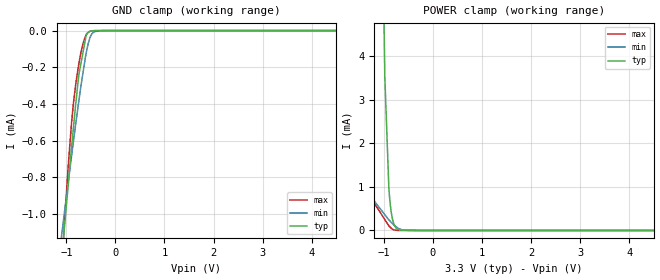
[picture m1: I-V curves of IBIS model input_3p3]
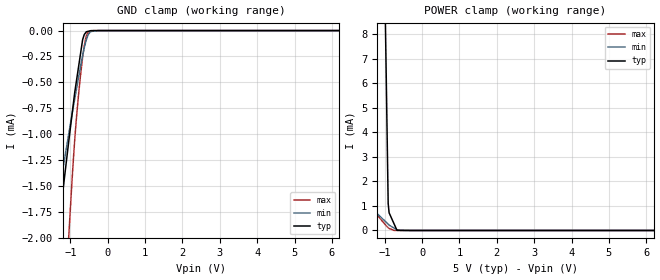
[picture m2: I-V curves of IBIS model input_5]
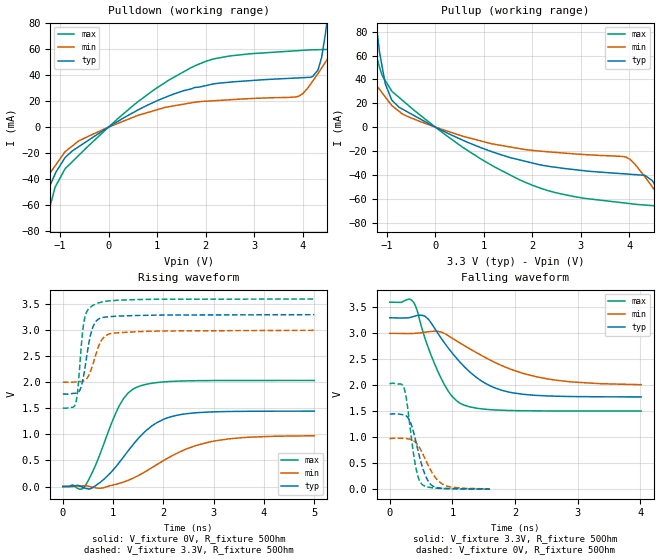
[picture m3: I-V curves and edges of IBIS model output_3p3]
|Texas Instruments Incorporated
| 10MHz Modulator with built in current excitation for Hall sensors
| Marketing part#   Digital Voltage Range   Package-type   #pins
| ADS1208IPW   2.7V - 5.5V   TSSOP   16
| ADS1208IPWG4   2.7V - 5.5V   TSSOP   16
| ADS1208IPWR   2.7V - 5.5V   TSSOP   16
| ADS1208IPWRG4   2.7V - 5.5V   TSSOP   16
[IBIS Ver]   3.2
[File name]   ads1208.ibs
|SIMDE Ver   V3.0 - 201101 - RHL4 - Build 457
[File Rev]   1.0
[Date]   5/16/2011
[Source]
| Texas Instruments Incorporated.
| Analog-eLab Design Center, HPA
| 12500 TI Blvd
| Dallas, TX -75243
| e-mail: elab_ibis@list.ti.com
[Notes]   Revision History:
| Rev 1.0: 5/16/2011
| - Initial version of the model
| - Model generated from simulations in TISPICE
| - Model matched to SPICE simulation
| - C_comp although listed in numerical order of value are
|   obtained from varying PVT conditions. For PVT conditions for
|   each specific value refer the buffer description under
|   respective [Model]. IBIS model user is responsible for using
|   appropriate C_comp to simulate for Signal Integrity.
| - Model names with a trailing _3p3 contains the model for
|   3.3V [3.0V and 3.6V]. Model names with a trailing _5 contains
|   the model for 5.0V [4.5V and 5.5V].
[Disclaimer]
| This model is designed as an aid for customers of Texas Instruments.
| TI and its licensors and suppliers make no warranties, either expressed
| or implied, with respect to this  model, including the warranties of
| merchantability or fitness for a particular purpose. The model is
| provided solely on an "as is" basis. The entire risk as to its quality
| and performance is with the customer.
[Copyright]
 (C) Copyright 2011 Texas Instruments Incorporated.All rights reserved.
|   ADS1208
[Component]   ADS1208
[Manufacturer]   TI
[Package]   |16 TSSOP   -  PW package
|   typ   min   max
R_pkg   0.03926   0.03631   0.04323
L_pkg   2.65777nH   2.30021nH   3.16884nH
C_pkg   0.46553pF   0.42516pF   0.51250pF
[Pin]  signal_name   model_name   R_pin   L_pin   C_pin
1   IOUT   TERM   0.03861   3.16884nH  0.51250pF
2   IADJ   TERM   0.04306   2.75459nH  0.48880pF
3   AVDD   POWER   0.02116   2.08677nH  0.46132pF
4   VIN+   TERM   0.03638   2.30226nH  0.43259pF
5   VIN-   TERM   0.03822   2.36501nH  0.43620pF
6   AGND   GND   0.02283   2.19557nH  0.46635pF
7   REFIN   TERM   0.04323   2.76940nH  0.48912pF
8   REFOUT   TERM   0.03809   3.16350nH  0.51239pF
9   M1   INPUT   0.03770   3.14936nH  0.51152pF
10   M0   INPUT   0.04232   2.73683nH  0.48790pF
11   _MDATA   OUTPUT   0.03883   2.39107nH  0.42516pF
12   MDATA   OUTPUT   0.03631   2.30021nH  0.42953pF
13   _MCLK   MCLK_BAR   0.03697   2.32042nH  0.43088pF
14   MCLK   OUTPUT   0.04145   2.47181nH  0.42976pF
15   BGND   GND   0.04286   2.74791nH  0.48822pF
16   BVDD   POWER   0.03789   3.14597nH  0.51159pF
|   Model Selectors
[Model Selector] INPUT
input_3p3  3.3V digital input
input_5   5.0V digital input
[Model Selector] OUTPUT
output_3p3  3.3V digital output
output_5   5.0V digital output
[Model Selector] MCLK_BAR
mclk_bar_3p3  3.3V digital I/O
mclk_bar_5   5.0V digital I/O
[Model Selector] TERM
term_3-3V  3.3V nominal termination
term_5-0V  5.0V nominal termination
[Model] term_3-3V
Model_type Terminator
C_comp   1.0e-20F  1.0e-20F  1.0e-20F
|   typ   min   max
[Voltage Range]   3.3V   3.0V   3.6V
[POWER Clamp Reference]   3.3V   3.0V   3.6V
[GND Clamp Reference]   0V   0V   0V
|Ambient Temperature   25   85   -40
|Junction Temperature
[Temperature Range]   35   95   -40
[Model] term_5-0V
Model_type Terminator
C_comp   1.0e-20F  1.0e-20F  1.0e-20F
|   typ   min   max
[Voltage Range]   5.0V   4.5V   5.5V
[POWER Clamp Reference]   5.0V   4.5V   5.5V
[GND Clamp Reference]   0V   0V   0V
|Ambient Temperature   25   85   -40
|Junction Temperature
[Temperature Range]   35   95   -40
| Models and submodels in the file (8): input_3p3 (Input), input_5 (Input), output_3p3 (Output), output_5 (Output), mclk_bar_3p3 (I/O), mclk_bar_5 (I/O), term_3-3V (Terminator), term_5-0V (Terminator)
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|   input_3p3 Model
[Model]   input_3p3
Model_type   Input
Vinl = 0.8
Vinh = 2.0
|   typ   min   max
|   (nom PVT)   (fast PVT)   (slow PVT)
|C_comp from frequency sweep method (F=10MHz)
|Average
|C_comp   6.241e-13   5.507e-13   6.563e-13
|C_comp from LC tank measurement(L=1nH)
|Average
|Resonant Frequency(Hz)   5.262e+10   6.403e+10   7.720e+09
C_comp   9.157e-15   6.185e-15   4.254e-13
| Where nom  PVT is Nominal Process, 3.3V, 35C
|   Fast PVT is Strong Process,  3.6V, -40C
|   Slow PVT is Weak Process,   3V, 95C
[Voltage Range]   3.3   3   3.6
|Ambient Temperature   25   85   -40
|Junction Temperature
[Temperature Range]   35   95   -40
[Power Clamp Reference]   3.3   3   3.6
[GND Clamp Reference]   0   0   0
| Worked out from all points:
|   GND clamp passes 1 mA (typ) near -1.01 V on its own axis
|   POWER clamp passes 1 mA (typ) near -0.90 V on its own axis
[GND Clamp]
|   Voltage   I(typ)   I(min)   I(max)
-3.3V     -8.305mA   -6.084mA   -13.52mA
-1.188V   -1.522mA   -1.315mA   -1.706mA
-1.048V   -1.099mA   -1.01mA    -1.087mA
-896.4mV  -643.4uA   -689uA     -511.2uA
-813.6mV  -412.9uA   -518.6uA   -302.1uA
-745.8mV  -241.2uA   -385.3uA   -182.8uA
-658.8mV  -116.1uA   -227uA     -69.11uA
-590.7mV  -18.21uA   -115.8uA   -22.97uA
-534.6mV  -5.388uA   -52.7uA    -6.77uA
-429mV    -393nA     -5.602uA   -329.7nA
-285mV    -260.1nA   -127.2nA   -169.2nA
6.6V      0A         0A         0A
[POWER Clamp]
|   Voltage   I(typ)   I(min)   I(max)
-3.3V     1.038A     4.406mA    5.171mA
-3V       885.5mA    3.863mA    4.508mA
-1.386V   105.8mA    991.9uA    1.005mA
-1.04V    8.055mA    448.9uA    354.1uA
-980.1mV  3.535mA    362.7uA    249.8uA
-897.6mV  969.7uA    243.1uA    104.9uA
-867.9mV  585uA      208.4uA    71.07uA
-851.4mV  436.9uA    189.2uA    52.7uA
-806.4mV  190.1uA    136.9uA    19.42uA
-745.8mV  50.64uA    82uA       5.864uA
-666.6mV  6.537uA    30.76uA    434.9nA
6.6V      0A         0A         0A
|   input_5 Model
[Model]   input_5
Model_type   Input
Vinl = 1.5
Vinh = 3.5
|   typ   min   max
|   (nom PVT)   (fast PVT)   (slow PVT)
|C_comp from frequency sweep method (F=10MHz)
|Average
|C_comp   5.579e-13   4.948e-13   6.238e-13
|C_comp from LC tank measurement(L=1nH)
|Average
|Resonant Frequency(Hz)   5.197e+10   6.383e+10   8.320e+09
C_comp   9.388e-15   6.223e-15   3.663e-13
| Where nom  PVT is Nominal Process, 5V, 35C
|   Fast PVT is Strong Process,  5.5V, -40C
|   Slow PVT is Weak Process,   4.5V, 95C
[Model Spec]
|Subparameter   typ   min   max
Vinh   3.5   3.15   3.85
Vinl   1.5   1.35   1.65
[Voltage Range]   5   4.5   5.5
|Ambient Temperature   25   85   -40
|Junction Temperature
[Temperature Range]   35   95   -40
[Power Clamp Reference]   5   4.5   5.5
[GND Clamp Reference]   0   0   0
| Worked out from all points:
|   GND clamp passes 1 mA (typ) near -1.02 V on its own axis
|   POWER clamp passes 1 mA (typ) near -0.90 V on its own axis
[GND Clamp]
|   Voltage   I(typ)   I(min)   I(max)
-5V       -13.84mA   -9.976mA   -29.85mA
-1.601V   -2.825mA   -2.233mA   -5.783mA
-1.373V   -2.099mA   -1.722mA   -4.208mA
-1.188V   -1.523mA   -1.315mA   -2.955mA
-1.045V   -1.083mA   -1.007mA   -2.016mA
-880mV    -596.4uA   -660.7uA   -1.053mA
-786.5mV  -371.2uA   -471.3uA   -650.6uA
-670mV    -90.54uA   -243uA     -260.2uA
-570mV    -11.61uA   -88.91uA   -51.87uA
-454.5mV  -1.103uA   -9.818uA   -7.056uA
-252mV    -268.3nA   -46.33nA   -34.87nA
10V       0A         0A         0A
[POWER Clamp]
|   Voltage   I(typ)   I(min)   I(max)
-5V       1.912A     7.552mA    8.964mA
-4.5V     1.654A     6.628mA    7.863mA
-1.665V   227.4mA    1.468mA    1.621mA
-1.375V   101.4mA    973.6uA    982.5uA
-1.14V    24.49mA    602.2uA    522.2uA
-957mV    6.273mA    335.6uA    189.5uA
-905mV    1.096mA    259.8uA    114.2uA
-880mV    720.8uA    223.4uA    82.72uA
-748mV    272.3uA    98.92uA    2.991uA
-670mV    7.189uA    29.51uA    2.679uA
-435mV    0A         3.245uA    1.739uA
10V       0A         0A         0A
|   output_3p3 Model
[Model]   output_3p3
Model_type   Output
Polarity   Non-Inverting
Vmeas = 1.65
Vref = 1.65
Cref = 30pF
Rref = 50
|   typ   min   max
|   (nom PVT)   (fast PVT)   (slow PVT)
|C_comp from frequency sweep method (F=10MHz)
|C_comp   2.140e-12   2.125e-12   2.174e-12
|ON state : BUFFER OUTPUT TURNED HIGH
|C_comp   2.140e-12   2.125e-12   2.174e-12
|OFF state: BUFFER OUTPUT TURNED LOW
|C_comp   2.055e-12   1.892e-12   2.087e-12
|C_comp from LC tank measurement(L=1nH)
|Resonant Frequency(Hz)   5.890e+09   6.040e+09   4.920e+09
C_comp   7.309e-13   6.950e-13   1.047e-12
|ON state : BUFFER OUTPUT TURNED HIGH
|Resonant Frequency(Hz)   5.890e+09   6.040e+09   4.920e+09
|C_comp   7.309e-13   6.950e-13   1.047e-12
|OFF state: BUFFER OUTPUT TURNED LOW
|Resonant Frequency(Hz)   5.960e+09   6.210e+09   5.000e+09
|C_comp   7.138e-13   6.575e-13   1.014e-12
| Where nom  PVT is Nominal Process, 3.3V, 35C
|   Fast PVT is Strong Process,  3.6V, -40C
|   Slow PVT is Weak Process,   3V, 95C
[Voltage Range]   3.3   3   3.6
|Ambient Temperature   25   85   -40
|Junction Temperature
[Temperature Range]   35   95   -40
[Pullup Reference]   3.3   3   3.6
[Pulldown Reference]   0   0   0
[Power Clamp Reference]   3.3   3   3.6
[GND Clamp Reference]   0   0   0
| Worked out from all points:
|   slope of the pulldown table from 0 to 0.495 V, typ, clamps not added: 45.5 ohm
|   slope of the pullup table from 0 to 0.495 V, typ, clamps not added: 51.2 ohm
|   falling waveform, V_fixture 3.3V, R_fixture 50Ohm: 20-80 % time 696ps typ, 1.05ns min, 421ps max; typ from 3.3 V to 1.78 V
|   rising waveform, V_fixture 0V, R_fixture 50Ohm: 20-80 % time 789ps typ, 1.15ns min, 521ps max; typ from 0 V to 1.45 V
|   rising waveform, V_fixture 3.3V, R_fixture 50Ohm: 20-80 % time 170ps typ, 217ps min, 120ps max; typ from 1.78 V to 3.3 V
|   falling waveform, V_fixture 0V, R_fixture 50Ohm: 20-80 % time 193ps typ, 260ps min, 140ps max; typ from 1.45 V to 0.004 V
[Pulldown]
|   Voltage   I(typ)   I(min)   I(max)
-3.3V     -235.7mA   -157.4mA   -409.3mA
-2.239V   -138.2mA   -94.86mA   -228.4mA
-1.494V   -69.65mA   -50.91mA   -104.6mA
-1.339V   -56.04mA   -42.39mA   -79.85mA
-896.4mV  -23.44mA   -18.92mA   -32.04mA
1.804V    30.54mA    19.28mA    47.49mA
3.918V    37.83mA    23.71mA    58.78mA
4.316V    43.89mA    41.12mA    59.47mA
4.496V    79.66mA    51.4mA     59.66mA
4.77V     187.5mA    67.5mA     62.15mA
4.918V    256.1mA    76.32mA    77.72mA
6.6V      1.096A     178.4mA    358.6mA
[Pullup]
|   Voltage   I(typ)   I(min)   I(max)
-3.3V     1.096A     160mA      409.7mA
-2.148V   510.7mA    90.38mA    215.2mA
-1.482V   191.2mA    50.08mA    102.7mA
-1.294V   112mA      39.22mA    71.39mA
-1.033V   36.28mA    25.3mA     38.94mA
-745.8mV  16.6mA     13.14mA    24.8mA
1.836V    -28.44mA   -18.71mA   -45.95mA
3.933V    -39.25mA   -25.19mA   -63.72mA
4.468V    -44.78mA   -49.97mA   -65.74mA
4.975V    -86.86mA   -79.66mA   -88.67mA
5.069V    -94.78mA   -85.15mA   -102.6mA
6.6V      -235.9mA   -175.1mA   -358.1mA
[Ramp]
R_load = 50
|   typ   min   max
dV/dt_r   0.868601/7.88674e-10   0.584928/1.15225e-09   1.22229/5.19124e-10
dV/dt_f   0.914229/6.96224e-10   0.596986/1.06545e-09   1.25642/4.21049e-10
[Falling Waveform]
V_fixture = 3.3V
V_fixture_min = 3V
V_fixture_max = 3.6V
R_fixture = 50Ohm
|   Time   V(typ)   V(min)   V(max)
0s        3.3V       3V         3.6V
378ps     3.323V     2.999V     3.602V
570ps     3.322V     3.023V     2.877V
820ps     2.908V     3.025V     2.135V
998ps     2.62V      2.906V     1.784V
1.185ns   2.365V     2.768V     1.62V
1.534ns   2.033V     2.529V     1.539V
1.962ns   1.856V     2.296V     1.514V
2.637ns   1.791V     2.101V     1.507V
4.013ns   1.777V     2.013V     1.506V
[Rising Waveform]
V_fixture = 0V
V_fixture_min = 0V
V_fixture_max = 0V
R_fixture = 50Ohm
|   Time   V(typ)   V(min)   V(max)
0s        687.6pV    1.215nV    632.9pV
416ps     -23.24mV   15.6mV     -22.5mV
737ps     75.12mV    -34.09mV   616.1mV
1.124ns   464.2mV    60.16mV    1.554V
1.291ns   676.1mV    115.9mV    1.788V
1.491ns   913.6mV    205.3mV    1.915V
1.881ns   1.232V     427.9mV    1.998V
2.35ns    1.383V     676.9mV    2.026V
3.296ns   1.441V     914.7mV    2.036V
4.999ns   1.448V     974.9mV    2.037V
[Rising Waveform]
V_fixture = 3.3V
V_fixture_min = 3V
V_fixture_max = 3.6V
R_fixture = 50Ohm
|   Time   V(typ)   V(min)   V(max)
0s        1.776V     2.003V     1.506V
253ps     1.791V     2.01V      1.589V
294ps     1.801V     2.013V     1.837V
345ps     1.865V     2.017V     2.43V
433ps     2.242V     2.036V     3.228V
548ps     2.9V       2.207V     3.441V
668ps     3.182V     2.571V     3.511V
798ps     3.247V     2.85V      3.549V
972ps     3.265V     2.942V     3.57V
4.999ns   3.3V       3V         3.6V
[Falling Waveform]
V_fixture = 0V
V_fixture_min = 0V
V_fixture_max = 0V
R_fixture = 50Ohm
|   Time   V(typ)   V(min)   V(max)
0s        1.448V     978.5mV    2.037V
230ps     1.43V      977.4mV    1.94V
272ps     1.403V     973.2mV    1.691V
331ps     1.287V     961.7mV    1.135V
411ps     952.2mV    904.4mV    455.3mV
468ps     661.5mV    815.5mV    183mV
519ps     431.4mV    702.8mV    89.62mV
649ps     99mV       377.8mV    34.13mV
845ps     18.29mV    97.03mV    13.78mV
1.595ns   4.095mV    6.884mV    1.723mV
